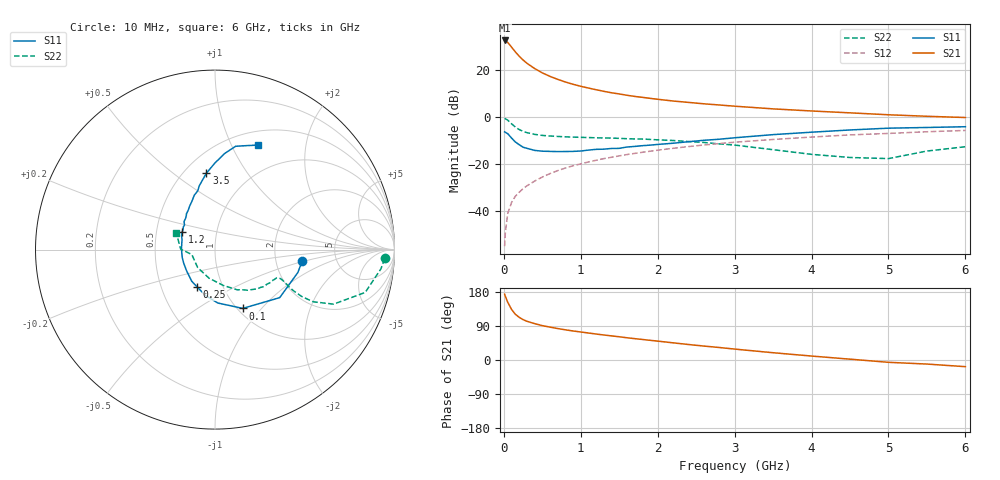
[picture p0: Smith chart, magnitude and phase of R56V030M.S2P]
! SIEMENS Small Signal Semiconductors
! BFR183
! Si NPN RF Bipolar Junction Transistor in SOT23
! VCE = 6 V  IC = 30 mA
! Common Emitter S-Parameters:  May  1996
# GHz  S  MA  R  50
!  f  S11  S21  S12  S22
! GHz  MAG  ANG  MAG  ANG  MAG  ANG  MAG  ANG
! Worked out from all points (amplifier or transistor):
!   36 points, 10 MHz to 6 GHz, reference 50 ohm
!   highest |S21| = 32.7 dB at 10 MHz (marker M1)
!   |S21| within 3 dB of that: start of sweep to 104.3 MHz
!   unconditionally stable (mu >= 1): 475.2 MHz to 2.407 GHz
!   at 250 MHz: K = 0.87, MSG = 27.4 dB, |S12| = -30.4 dB
!   at 1.4 GHz: K = 1.04, MAG = 12.5 dB, |S12| = -17.0 dB
!   at 6 GHz: K = 0.90, MSG = 2.8 dB, |S12| = -5.6 dB
!   S11 on the Smith chart (normalised r, x): 10 MHz: 2.82, -0.49; 100 MHz: 1.06, -0.80; 250 MHz: 0.76, -0.33; 1.2 GHz: 0.68, +0.14; 3.5 GHz: 0.64, +0.66; 6 GHz: 0.66, +1.27
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0.01  0.4894 -7.7  43.36 173.6  0.0018 87.4  0.9465 -3.0
0.02  0.4791 -15.4  42.97 167.9  0.0036 85.4  0.9309 -6.6
0.05  0.449 -36.6  39.45 152.6  0.0088 77.6  0.8704 -15.9
0.1  0.3621 -64.8  31.33 133.6  0.0153 72.7  0.7272 -24.7
0.15  0.2979 -87.0  24.7 120.6  0.0209 69.3  0.619 -28.0
0.2  0.261 -101.7  20.02 112.5  0.0253 70.4  0.5486 -28.4
0.25  0.2308 -115.5  16.63 106.6  0.0302 70.3  0.5017 -27.8
0.3  0.2187 -126.4  14.18 102.2  0.0347 71.7  0.4711 -27.1
0.4  0.1974 -143.5  10.95 96.0  0.0438 73.2  0.4335 -25.3
0.5  0.1899 -156.6  8.846 90.7  0.0534 73.2  0.4115 -24.3
0.6  0.188 -165.8  7.445 86.7  0.0633 73.4  0.3998 -23.9
0.7  0.186 -175.3  6.439 83.0  0.0732 73.0  0.3912 -24.0
0.8  0.1868 177.2  5.651 79.6  0.0831 72.5  0.3842 -24.2
0.9  0.188 170.0  5.054 76.6  0.0929 71.9  0.3789 -24.6
1.1  0.2003 158.1  4.2 71.2  0.112 70.5  0.3705 -26.7
1.2  0.2078 152.5  3.871 68.5  0.1217 69.5  0.3661 -27.6
1.6  0.233 137.7  2.95 58.7  0.161 65.5  0.35 -33.0
2.2  0.2805 120.2  2.225 45.3  0.2187 58.9  0.3208 -43.0
3.5  0.4279 96.5  1.513 19.2  0.3374 42.3  0.2044 -77.2
4.5  0.5378 84.3  1.245 2.2  0.4223 29.7  0.1394 -133.7
5.5  0.6074 72.6  1.052 -10.7  0.4926 18.2  0.1912 179.3
6  0.6302 67.5  0.99 -17.6  0.5253 10.7  0.2364 156.3
